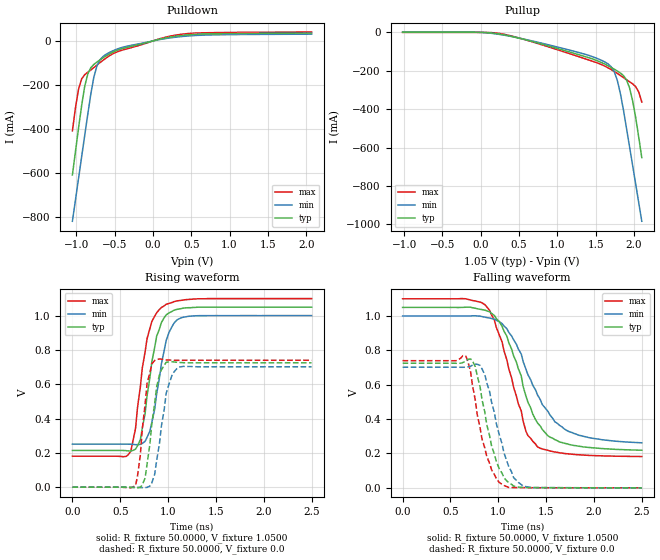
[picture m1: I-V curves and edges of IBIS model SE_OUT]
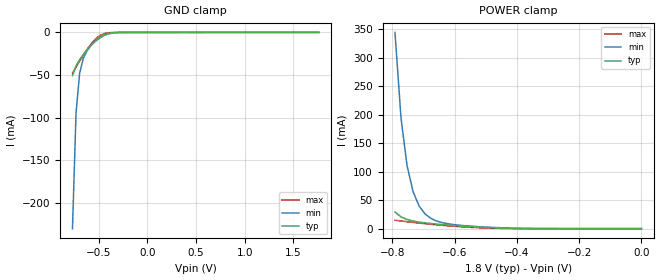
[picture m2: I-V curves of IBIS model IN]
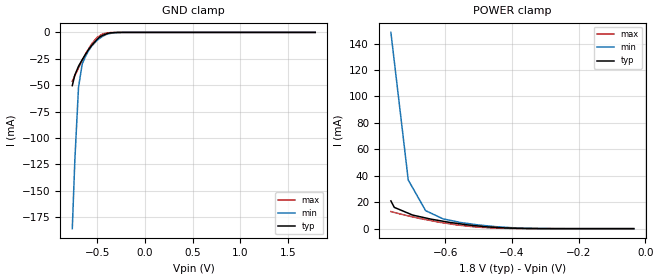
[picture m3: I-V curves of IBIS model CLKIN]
| Integrated Devices Technolgy, Inc
[IBIS Ver]   4.2
[File name]   9sbv0802.ibs
[File Rev]   1.3
|Rev history   1.3   2016-05-04 fix typo in pin 8 signal name
|Rev history   1.2   12-09 update SE_OUT data
|Rev history   1.1   08-13 update CLKIN data
|Rev history   1.0   original revision
[Date]   4 May, 2016
[Disclaimer] Integrated Device Technology, Inc. ("IDT") hereby grants the
   user of this ibis model a non-exclusive, nontransferable
   license to use this ibis model under the following terms. the
   user is granted this license only to use the ibis model and is
   not granted rights to sell, copy (except as needed to run the
   ibis model), rent, lease or sub-license the ibis model in
   whole or in part, or in modified form to anyone. the user may
   modify the ibis model to suit its specific applications, but
   rights to derivative works and such modifications shall belong
   to idt. this ibis model is provided on an as is" basis and idt
   makes absolutely no warranty with respect to the information
   contained herein. idt disclaims and customer waives all
   warranties, express and implied, including warranties of
   merchantability and fitness for a particular purpose. the
   entire risk as to quality and performance is with the user
   accordingly, in no event shall idt be liable for any direct or
   indirect damages, whether in contract or tort, including any
   lost profits or other incidental, consequential, exemplary, or
   punitive damages arising out of the use or application of the
   ibis model. further, idt reserves the right to make changes
   without notice to any product herein to improve reliability,
   function, or design. idt does not convey any license under
   patent rights or any other intellectual property rights,
   including those of third parties. idt is not obligated to
   provide maintenance or support for the licensed ibis model.
[Copyright]   Copyright 2012, Integrated Devices Technolgy, Inc. all rights
   reserved
[Component]   9SBV0802
[Manufacturer] Integrated Device Technology, Inc.
[Package]
R_pkg   72.4655m   58.886m   86.045m
L_pkg   1.47175nH   1.11650nH   1.77850nH
C_pkg   0.07747pF   0.07444pF   0.08050pF
[Pin] signal_name  model_name
1 VDD1.8   POWER
2 ICLKA_1.05   CLKIN
3 VREF_1.05   CLKIN
4 ICLKB_1.05   CLKIN
5 VDD1.8   POWER
6 Q_7   SE_OUT
7 VDD1.8   POWER
8 Q_6   SE_OUT
9 vOE_16#   IN
10 Q_5   SE_OUT
11 VDDD1.8   POWER
12 Q_4   SE_OUT
13 vOE2345#   IN
14 Q_3   SE_OUT
15 VDD1.8   POWER
16 Q_2   SE_OUT
17 vOE07#   IN
18 Q_1   SE_OUT
19 VDD1.8   POWER
20 Q_0   SE_OUT
21 EPAD   GND
| Models and submodels in the file (3): SE_OUT (Output), IN (Input), CLKIN (Input)
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|   Model SE_OUT
[Model]  SE_OUT
Model_type Output
Polarity   Non-Inverting
Enable   Active-High
Vmeas =  0.5000V
Cref =   2.0000pF
Rref =   0.0
Vref =   0.5000V
C_comp   1.1000pF   1.0000pF   1.2000pF
[Temperature Range]   25.0000   100.0000   -40.0000
[Voltage Range]   1.0500V   1.0000V   1.1000V
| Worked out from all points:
|   slope of the pulldown table from 0 to 0.158 V, typ, clamps not added: 12.1 ohm
|   slope of the pullup table from 0 to 0.158 V, typ, clamps not added: 40.1 ohm
|   rising waveform, R_fixture 50.0000, V_fixture 1.0500: 20-80 % time 139ps typ, 139ps min, 142ps max; typ from 0.214 V to 1.05 V
|   rising waveform, R_fixture 50.0000, V_fixture 0.0: 20-80 % time 96.2ps typ, 112ps min, 77.8ps max; typ from 0 V to 0.725 V
|   falling waveform, R_fixture 50.0000, V_fixture 1.0500: 20-80 % time 314ps typ, 391ps min, 279ps max; typ from 1.05 V to 0.219 V
|   falling waveform, R_fixture 50.0000, V_fixture 0.0: 20-80 % time 174ps typ, 191ps min, 173ps max; typ from 0.725 V to 0 V
[Pulldown]
|Voltage   I(typ)   I(min)   I(max)
-1.05V    -607.7mA   -817.8mA   -407.8mA
-1.01V    -500.9mA   -720.5mA   -302.9mA
-970mV    -394.9mA   -623.4mA   -219.3mA
-930mV    -294.3mA   -526.5mA   -172.7mA
-890mV    -206.9mA   -429.8mA   -153.2mA
-850mV    -150.2mA   -333.7mA   -142mA
-770mV    -106.5mA   -163.6mA   -120.8mA
-730mV    -95.56mA   -113.1mA   -109.5mA
-650mV    -76.55mA   -70.17mA   -87.48mA
-370mV    -31.87mA   -26.48mA   -38.68mA
350mV     23.67mA    19mA       29.26mA
2.07V     35.48mA    30.76mA    40.31mA
[Pullup]
|Voltage   I(typ)   I(min)   I(max)
-1.02V    473.8uA    1.851mA    50.9uA
260mV     -9.719mA   -11.52mA   -6.584mA
1.3V      -118.8mA   -107.1mA   -129.4mA
1.66V     -173.9mA   -164.3mA   -184.5mA
1.74V     -191.6mA   -204.2mA   -203.3mA
1.78V     -201.1mA   -248.7mA   -213.6mA
1.86V     -224.6mA   -402.4mA   -235.4mA
1.94V     -288.8mA   -595.2mA   -257.1mA
1.98V     -355.7mA   -692.2mA   -268.1mA
2.02V     -442.7mA   -789.5mA   -282.4mA
2.06V     -545.8mA   -886.8mA   -310.4mA
2.1V      -652.6mA   -984.3mA   -362.8mA
[Ramp]
| variable   typ   min   max
dV/dt_r  0.4350/96.4252p   0.4211/0.1112n   0.4439/80.7075p
dV/dt_f  0.4987/0.3416n   0.4427/0.4090n   0.5507/0.2917n
R_load = 50.0000
[Rising Waveform]
R_fixture= 50.0000
V_fixture= 1.0500
V_fixture_min= 1.0000
V_fixture_max= 1.1000
|time   V(typ)   V(min)   V(max)
0s        214.2mV    251mV      180.7mV
560ps     213.2mV    251.1mV    179.6mV
610ps     211mV      250.5mV    208.9mV
660ps     221.9mV    248.3mV    343.1mV
710ps     276.3mV    249.7mV    583.8mV
780ps     532.6mV    290.5mV    865mV
880ps     878.7mV    542.5mV    1.016V
980ps     1.004V     855.3mV    1.066V
1.21ns    1.046V     995.7mV    1.094V
2.5ns     1.049V     1V         1.099V
[Rising Waveform]
R_fixture= 50.0000
V_fixture= 0.0
V_fixture_min= 0.0
V_fixture_max= 0.0
|time   V(typ)   V(min)   V(max)
0s        0V         597.7nV    0V
660ps     -3.079mV   142.6uV    9.928mV
710ps     -915.2uV   -1.443mV   188.9mV
760ps     53.54mV    -2.379mV   484.5mV
780ps     133.3mV    -959.1uV   603.7mV
830ps     370.5mV    25.11mV    718.4mV
880ps     584.2mV    154.2mV    745.1mV
980ps     728mV      546.7mV    741.8mV
1.11ns    727.1mV    699.4mV    739.4mV
2.5ns     725mV      701.8mV    739.9mV
[Falling Waveform]
R_fixture= 50.0000
V_fixture= 1.0500
V_fixture_min= 1.0000
V_fixture_max= 1.1000
|time   V(typ)   V(min)   V(max)
0s        1.05V      1V         1.1V
860ps     1.034V     993.2mV    1.066V
960ps     1.002V     981.5mV    974.6mV
1.09ns    882.3mV    925.8mV    744.2mV
1.24ns    651.2mV    779.1mV    448.1mV
1.29ns    532.1mV    688.8mV    327.7mV
1.41ns    377.8mV    540.7mV    237.9mV
1.59ns    280.9mV    384.8mV    208.7mV
1.74ns    252.4mV    327.2mV    197.1mV
2.5ns     218.9mV    262.1mV    182.2mV
[Falling Waveform]
R_fixture= 50.0000
V_fixture= 0.0
V_fixture_min= 0.0
V_fixture_max= 0.0
|time   V(typ)   V(min)   V(max)
0s        725.1mV    701.8mV    739.9mV
660ps     737.3mV    701.9mV    767.2mV
710ps     750.3mV    707.5mV    677.2mV
760ps     704.6mV    719.1mV    509.3mV
860ps     439mV      657.8mV    230.6mV
930ps     243.9mV    498.4mV    104.9mV
1.06ns    59mV       202.4mV    13.67mV
1.16ns    10.27mV    59.49mV    1.769mV
1.26ns    1.914mV    10.62mV    1.139mV
2.5ns     94.06uV    197.8uV    42.59uV
|   Model IN
[Model]   IN
Model_type   Input
Polarity   Non-Inverting
Vinl = 0.63V
Vinh = 1.17V
|   typ   min   max
C_comp   2pF   1.5pF   2.5pF
|   typ   min   max
[Voltage range]   1.8V   1.7V   1.9V
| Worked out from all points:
|   GND clamp passes 1 mA (typ) near -0.39 V on its own axis
|   POWER clamp passes 1 mA (typ) near -0.45 V on its own axis
[GND_clamp]
|Voltage   I (typ)   I (min)   I (max)
|Note, modeling breaks down at 250mA and above.  This is well beyond the functional   |
|operating range of the device.  Should this scenario occur, catastrophic failure and   |
|possible damage to the device and/or board is of higher concern than the I-V curve   |
|behavior.  The IBIS checker will flag currents in excess of 10A with warnings.  Lines   |
|with currents in excess of 0.35 A have been commented out.  The points still remain|
|available to the user if the user desires to use them.   |
|-1.80000e+00   -4.43726e+01   -4.17458e+01   -4.86820e+01
|-1.76327e+00   -4.25922e+01   -4.02056e+01   -4.65395e+01
|-1.72653e+00   -4.08117e+01   -3.86654e+01   -4.43969e+01
|-1.68980e+00   -3.90312e+01   -3.71251e+01   -4.22544e+01
|-1.65306e+00   -3.72507e+01   -3.55849e+01   -4.01118e+01
|-1.61633e+00   -3.54702e+01   -3.40446e+01   -3.79693e+01
|-1.57959e+00   -3.36896e+01   -3.25043e+01   -3.58267e+01
|-1.54286e+00   -3.19091e+01   -3.09640e+01   -3.36840e+01
|-1.50612e+00   -3.01285e+01   -2.94236e+01   -3.15414e+01
|-1.46939e+00   -2.83479e+01   -2.78833e+01   -2.93987e+01
|-1.43265e+00   -2.65672e+01   -2.63429e+01   -2.72561e+01
|-1.39592e+00   -2.47866e+01   -2.48025e+01   -2.51134e+01
|-1.35918e+00   -2.30059e+01   -2.32621e+01   -2.29707e+01
|-1.32245e+00   -2.12253e+01   -2.17217e+01   -2.08279e+01
|-1.28571e+00   -1.94446e+01   -2.01813e+01   -1.86852e+01
|-1.24898e+00   -1.76639e+01   -1.86409e+01   -1.65424e+01
|-1.21224e+00   -1.58832e+01   -1.71005e+01   -1.43996e+01
|-1.17551e+00   -1.41025e+01   -1.55600e+01   -1.22568e+01
|-1.13878e+00   -1.23218e+01   -1.40196e+01   -1.01141e+01
|-1.10204e+00   -1.05411e+01   -1.24792e+01   -7.97124e+00
|-1.06531e+00   -8.76046e+00   -1.09388e+01   -5.82843e+00
|-1.02857e+00   -6.97978e+00   -9.39848e+00   -3.68562e+00
|-9.91837e-01   -5.19912e+00   -7.85813e+00   -1.54785e+00
|-9.55102e-01   -3.41847e+00   -6.31781e+00   -3.90595e-01
|-9.18367e-01   -1.63807e+00   -4.77753e+00   -1.29996e-01
|-8.81633e-01   -5.21907e-01   -3.23728e+00   -7.87800e-02
|-8.44898e-01   -1.73459e-01   -1.69709e+00   -6.40873e-02
|-8.08163e-01   -7.85613e-02   -6.33127e-01   -5.54276e-02
-771.4mV  -50.63mA   -230.2mA   -47.85mA
-734.7mV  -39.27mA   -94.07mA   -40.58mA
-698mV    -32.06mA   -48.05mA   -33.55mA
-661.2mV  -26.07mA   -30.55mA   -26.83mA
-624.5mV  -20.62mA   -22.01mA   -20.51mA
-587.8mV  -15.64mA   -16.46mA   -14.75mA
-514.3mV  -7.457mA   -8.514mA   -5.771mA
-477.6mV  -4.509mA   -5.592mA   -2.97mA
-404.1mV  -1.167mA   -1.846mA   -517.4uA
-293.9mV  -74.63uA   -181.5uA   -23.43uA
1.763V    14.13uA    10.16uA    21.47uA
[Power_clamp]
|Voltage   I (typ)   I (min)   I (max)
|Note, modeling breaks down at 250mA and above.  This is well beyond the functional   |
|operating range of the device.  Should this scenario occur, catastrophic failure and   |
|possible damage to the device and/or board is of higher concern than the I-V curve   |
|behavior.  The IBIS checker will flag currents in excess of 10A with warnings.  Lines   |
|with currents in excess of 0.35 A have been commented out.  The points still remain|
|available to the user if the user desires to use them.   |
|-1.80000e+00   5.60662e+01   5.31750e+01   6.07752e+01
|-1.78061e+00   5.48637e+01   5.21252e+01   5.93477e+01
|-1.76122e+00   5.36611e+01   5.10754e+01   5.79201e+01
|-1.74184e+00   5.24586e+01   5.00255e+01   5.64925e+01
|-1.72245e+00   5.12561e+01   4.89757e+01   5.50649e+01
|-1.70306e+00   5.00535e+01   4.79259e+01   5.36374e+01
|-1.68367e+00   4.88510e+01   4.68761e+01   5.22098e+01
|-1.66429e+00   4.76485e+01   4.58263e+01   5.07822e+01
|-1.64490e+00   4.64460e+01   4.47765e+01   4.93547e+01
|-1.62551e+00   4.52434e+01   4.37267e+01   4.79271e+01
|-1.60612e+00   4.40409e+01   4.26769e+01   4.64996e+01
|-1.58673e+00   4.28384e+01   4.16272e+01   4.50720e+01
|-1.56735e+00   4.16359e+01   4.05774e+01   4.36444e+01
|-1.54796e+00   4.04334e+01   3.95276e+01   4.22169e+01
|-1.52857e+00   3.92308e+01   3.84778e+01   4.07893e+01
|-1.50918e+00   3.80283e+01   3.74280e+01   3.93618e+01
|-1.48980e+00   3.68258e+01   3.63783e+01   3.79342e+01
|-1.47041e+00   3.56233e+01   3.53285e+01   3.65067e+01
|-1.45102e+00   3.44208e+01   3.42787e+01   3.50791e+01
|-1.43163e+00   3.32183e+01   3.32290e+01   3.36516e+01
|-1.41224e+00   3.20159e+01   3.21792e+01   3.22241e+01
|-1.39286e+00   3.08134e+01   3.11294e+01   3.07965e+01
|-1.37347e+00   2.96109e+01   3.00797e+01   2.93690e+01
|-1.35408e+00   2.84084e+01   2.90300e+01   2.79415e+01
|-1.33469e+00   2.72059e+01   2.79802e+01   2.65140e+01
|-1.31531e+00   2.60035e+01   2.69305e+01   2.50865e+01
|-1.29592e+00   2.48010e+01   2.58808e+01   2.36589e+01
|-1.27653e+00   2.35986e+01   2.48310e+01   2.22314e+01
|-1.25714e+00   2.23961e+01   2.37813e+01   2.08039e+01
|-1.23776e+00   2.11937e+01   2.27316e+01   1.93764e+01
|-1.21837e+00   1.99912e+01   2.16819e+01   1.79490e+01
|-1.19898e+00   1.87888e+01   2.06322e+01   1.65215e+01
|-1.17959e+00   1.75864e+01   1.95825e+01   1.50940e+01
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-791.8mV  29.26mA    344.8mA    14.84mA
-772.4mV  20.73mA    194.3mA    13.49mA
-753.1mV  16.1mA     110.7mA    12.21mA
-733.7mV  13.35mA    64.84mA    10.99mA
-714.3mV  11.49mA    39.63mA    9.831mA
-694.9mV  10.08mA    25.65mA    8.721mA
-675.5mV  8.904mA    17.72mA    7.666mA
-636.7mV  6.907mA    10.16mA    5.729mA
-539.8mV  3.07mA     4.093mA    2.051mA
-365.3mV  167.9uA    383.5uA    57.09uA
0V        14.13nA    10.08nA    21.48nA
|   Model CLKIN
[Model]   CLKIN
Model_type   Input
Polarity   Non-Inverting
Vinl = 0.63V
Vinh = 1.17V
|   typ   min   max
C_comp   2pF   1.5pF   2.5pF
|   typ   min   max
[Voltage range]   1.8V   1.7V   1.9V
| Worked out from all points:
|   GND clamp passes 1 mA (typ) near -0.39 V on its own axis
|   POWER clamp passes 1 mA (typ) near -0.45 V on its own axis
[GND_clamp]
|Voltage   I (typ)   I (min)   I (max)
|Note, modeling breaks down at 250mA and above.  This is well beyond the functional   |
|operating range of the device.  Should this scenario occur, catastrophic failure and   |
|possible damage to the device and/or board is of higher concern than the I-V curve   |
|behavior.  The IBIS checker will flag currents in excess of 10A with warnings.  Lines   |
|with currents in excess of 0.35 A have been commented out.  The points still remain|
|available to the user if the user desires to use them.   |
|-1.84184e+00   -4.43726e+01   -3.75529e+01   -5.11219e+01
|-1.78367e+00   -4.35813e+01   -3.75529e+01   -4.77297e+01
|-1.72551e+00   -4.07622e+01   -3.75529e+01   -4.43374e+01
|-1.68980e+00   -3.90312e+01   -3.71251e+01   -4.22543e+01
|-1.64796e+00   -3.70034e+01   -3.53709e+01   -3.98142e+01
|-1.60918e+00   -3.51239e+01   -3.37451e+01   -3.75526e+01
|-1.57959e+00   -3.36896e+01   -3.25043e+01   -3.58266e+01
|-1.54388e+00   -3.19585e+01   -3.10067e+01   -3.37435e+01
|-1.49286e+00   -2.94854e+01   -2.88674e+01   -3.07676e+01
|-1.46939e+00   -2.83478e+01   -2.78832e+01   -2.93987e+01
|-1.43469e+00   -2.66661e+01   -2.64285e+01   -2.73750e+01
|-1.38776e+00   -2.43909e+01   -2.44602e+01   -2.46371e+01
|-1.35918e+00   -2.30059e+01   -2.32621e+01   -2.29706e+01
|-1.31837e+00   -2.10274e+01   -2.15505e+01   -2.05898e+01
|-1.28367e+00   -1.93456e+01   -2.00957e+01   -1.85661e+01
|-1.24898e+00   -1.76639e+01   -1.86409e+01   -1.65424e+01
|-1.20204e+00   -1.53885e+01   -1.66725e+01   -1.38044e+01
|-1.17959e+00   -1.43003e+01   -1.57312e+01   -1.24949e+01
|-1.13878e+00   -1.23218e+01   -1.40196e+01   -1.01140e+01
|-1.08571e+00   -9.74968e+00   -1.17946e+01   -7.01883e+00
|-1.07551e+00   -9.25505e+00   -1.13667e+01   -6.42361e+00
|-1.02755e+00   -6.93027e+00   -9.35566e+00   -3.62605e+00
|-9.73469e-01   -4.30875e+00   -7.08793e+00   -8.78143e-01
|-9.69388e-01   -4.11092e+00   -6.91679e+00   -6.70754e-01
|-9.18367e-01   -1.63803e+00   -4.77749e+00   -1.81535e-01
|-8.67347e-01   -3.93222e-01   -2.63828e+00   -7.78700e-02
|-8.53061e-01   -2.53802e-01   -2.12593e+00   -6.64177e-02
|-8.08163e-01   -7.85268e-02   -6.91421e-01   -5.57542e-02
-763.3mV  -50.4mA    -185.9mA   -46.26mA
-736.7mV  -40.46mA   -121.4mA   -40.95mA
-698mV    -32.04mA   -51.96mA   -33.61mA
-659.2mV  -25.86mA   -29.9mA    -26.57mA
-620.4mV  -20.15mA   -21.89mA   -19.82mA
-587.8mV  -15.62mA   -16.69mA   -14.97mA
-555.1mV  -11.83mA   -12.54mA   -10.4mA
-504.1mV  -6.773mA   -7.631mA   -4.854mA
-445.9mV  -2.89mA    -3.687mA   -1.475mA
-399mV    -1.185mA   -1.676mA   -541uA
-294.9mV  -85.59uA   -180.4uA   -23.42uA
1.787V    3.903nA    237nA      117.1pA
[Power_clamp]
|Voltage   I (typ)   I (min)   I (max)
|Note, modeling breaks down at 250mA and above.  This is well beyond the functional   |
|operating range of the device.  Should this scenario occur, catastrophic failure and   |
|possible damage to the device and/or board is of higher concern than the I-V curve   |
|behavior.  The IBIS checker will flag currents in excess of 10A with warnings.  Lines   |
|with currents in excess of 0.35 A have been commented out.  The points still remain|
|available to the user if the user desires to use them.   |
|-1.90000e+00   5.60662e+01   4.77602e+01   6.81385e+01
|-1.84184e+00   5.60662e+01   4.77602e+01   6.38558e+01
|-1.80000e+00   5.60662e+01   4.77602e+01   6.07752e+01
|-1.78367e+00   5.50536e+01   4.77602e+01   5.95731e+01
|-1.74490e+00   5.26485e+01   4.77602e+01   5.67179e+01
|-1.72551e+00   5.14459e+01   4.77602e+01   5.52904e+01
|-1.70000e+00   4.98637e+01   4.77602e+01   5.34120e+01
|-1.68980e+00   4.92308e+01   4.72076e+01   5.26606e+01
|-1.66735e+00   4.78384e+01   4.59921e+01   5.10076e+01
|-1.64796e+00   4.66358e+01   4.49423e+01   4.95801e+01
|-1.63469e+00   4.58130e+01   4.42240e+01   4.86033e+01
|-1.60918e+00   4.42308e+01   4.28427e+01   4.67250e+01
|-1.59592e+00   4.34080e+01   4.21244e+01   4.57482e+01
|-1.57959e+00   4.23954e+01   4.12404e+01   4.45461e+01
|-1.55102e+00   4.06232e+01   3.96933e+01   4.24423e+01
|-1.54388e+00   4.01802e+01   3.93066e+01   4.19163e+01
|-1.52449e+00   3.89777e+01   3.82568e+01   4.04888e+01
|-1.49286e+00   3.70157e+01   3.65440e+01   3.81596e+01
|-1.49184e+00   3.69524e+01   3.64888e+01   3.80845e+01
|-1.46939e+00   3.55600e+01   3.52732e+01   3.64316e+01
|-1.43980e+00   3.37247e+01   3.36710e+01   3.42527e+01
|-1.43469e+00   3.34082e+01   3.33947e+01   3.38770e+01
|-1.41429e+00   3.21424e+01   3.22897e+01   3.23743e+01
|-1.38776e+00   3.04969e+01   3.08532e+01   3.04209e+01
|-1.37653e+00   2.98008e+01   3.02455e+01   2.95944e+01
|-1.35918e+00   2.87249e+01   2.93062e+01   2.83172e+01
|-1.33571e+00   2.72692e+01   2.80355e+01   2.65891e+01
|-1.31837e+00   2.61933e+01   2.70962e+01   2.53119e+01
|-1.30408e+00   2.53073e+01   2.63228e+01   2.42600e+01
|-1.28367e+00   2.40416e+01   2.52178e+01   2.27574e+01
|-1.26020e+00   2.25860e+01   2.39471e+01   2.10293e+01
|-1.24898e+00   2.18898e+01   2.33393e+01   2.02029e+01
|-1.23163e+00   2.08139e+01   2.24001e+01   1.89257e+01
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-763.3mV  20.98mA    148.5mA    12.93mA
-753.1mV  16.09mA    126.6mA    12.25mA
-711.2mV  11.67mA    36.84mA    9.69mA
-698mV    10.27mA    30.93mA    8.925mA
-659.2mV  8.1mA      13.64mA    6.86mA
-607.1mV  5.621mA    7.447mA    4.453mA
-555.1mV  3.622mA    4.685mA    2.527mA
-451mV    999.8uA    1.546mA    418.9uA
-346.9mV  115.6uA    255.6uA    28.77uA
-34.69mV  5.354nA    84.02nA    174.7pA
